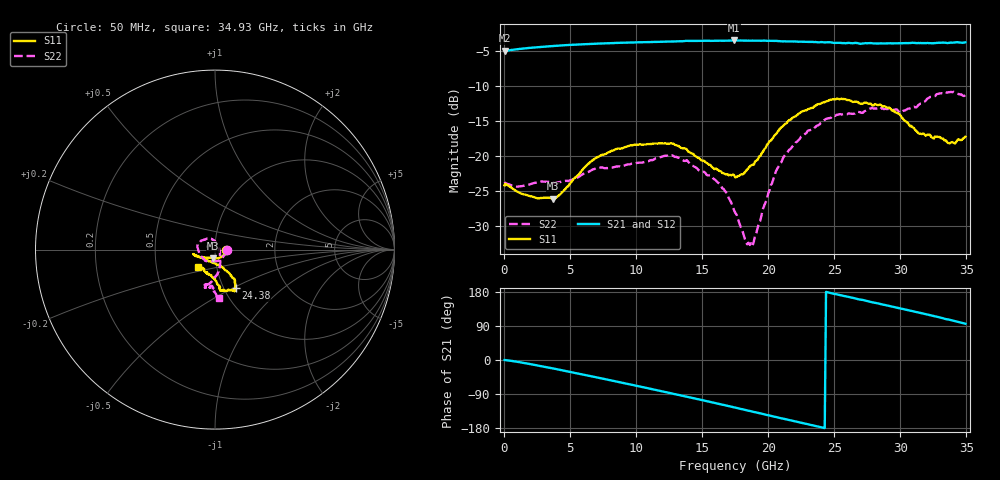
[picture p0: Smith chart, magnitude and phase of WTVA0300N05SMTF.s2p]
! 50 ohm 2-Port S-parameters measured by Modelithics Inc support@modelithics.com  Tampa, FL USA 813-866-6335 (February 2024)
! Smiths Interconnect,  3dB P/N: WTVA0300N05SMTF, Temperature: -50 C
! Board: 10 mil Rogers 4350B, Mounting Pad Dimensions: Length: 15 mils, Width: 25 mils, Gap: 40 mils.
# Hz S RI R 50
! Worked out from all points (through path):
!   352 points, 50 MHz to 34.93 GHz, reference 50 ohm
!   highest |S21| = -3.56 dB at 17.41 GHz (marker M1); lowest = -5.0 dB at 50 MHz (marker M2)
!   group delay of S21, straight-line fit = 21.4 ps
!   lowest |S11| = -26.1 dB at 3.683 GHz (marker M3), VSWR 1.10, Z = 48.6 - j4.69 ohm
!   |S11| at or under -10 dB: start of sweep to end of sweep
!   |S22| runs from -32.8 to -10.9 dB; largest |S21 - S12| = 0.0036
!   S11 on the Smith chart (normalised r, x): 50 MHz: 1.13, -0.01; 24.38 GHz: 1.13, -0.52; 34.93 GHz: 0.81, -0.16
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5e7  0.0617 -0.00236  0.5602 -0.00083  0.5602 -0.00124  0.0652 -0.00248
9.96e8  0.0453 -0.0326  0.5728 -0.0464  0.5727 -0.0464  0.0476 -0.0373
3.6825e9  -0.0123 -0.0482  0.561 -0.2276  0.5608 -0.2275  0.0065 -0.0639
5.8715e9  -0.0653 -0.0428  0.4938 -0.3798  0.4936 -0.3798  -0.0322 -0.0659
8.4585e9  -0.1063 -0.0347  0.3523 -0.5297  0.352 -0.5297  -0.0694 -0.0472
1.1742e10  -0.1205 -0.0254  0.1034 -0.6405  0.1028 -0.6404  -0.0971 0.00955
1.38315e10  -0.1062 -0.0343  -0.0766 -0.6553  -0.0767 -0.6552  -0.08 0.0482
1.56225e10  -0.0726 -0.0467  -0.2343 -0.616  -0.2346 -0.6156  -0.0351 0.0637
1.68165e10  -0.0453 -0.0586  -0.3316 -0.571  -0.332 -0.5707  -0.0101 0.0541
1.74135e10  -0.0317 -0.0658  -0.3801 -0.5438  -0.3802 -0.5437  0.00379 0.041
1.7513e10  -0.0273 -0.065  -0.3881 -0.5381  -0.3882 -0.5379  0.0045 0.0391
1.8309e10  -0.00013 -0.0782  -0.4448 -0.4906  -0.4447 -0.4906  0.0169 0.0176
1.88065e10  0.0146 -0.0852  -0.4773 -0.4587  -0.4771 -0.4585  0.0228 -0.000365
2.05975e10  0.0704 -0.125  -0.5743 -0.3235  -0.5745 -0.3227  0.0299 -0.0724
2.209e10  0.1053 -0.1605  -0.6219 -0.1973  -0.6218 -0.197  0.021 -0.1231
2.33835e10  0.1113 -0.1896  -0.642 -0.0826  -0.6418 -0.0825  -0.00297 -0.1534
2.43785e10  0.1147 -0.216  -0.6438 0.00408  -0.6437 0.00417  -0.0228 -0.182
2.91545e10  0.0253 -0.2194  -0.5032 0.3846  -0.5029 0.3848  -0.0325 -0.214
3.005e10  0.0125 -0.1913  -0.4542 0.4412  -0.454 0.4412  -0.0169 -0.2024
3.1443e10  -0.0207 -0.1428  -0.3637 0.5212  -0.3633 0.5213  -0.00682 -0.233
3.3632e10  -0.0598 -0.1079  -0.1859 0.6086  -0.183 0.6093  0.0377 -0.2815
3.49255e10  -0.0947 -0.0991  -0.0644 0.6402  -0.0621 0.6403  0.0218 -0.2696
